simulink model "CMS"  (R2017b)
settings: Solver=FixedStepDiscrete  StartTime=0.0  StopTime=10.0  FixedStep=0.01  RelTol=1e-3  EnableMultiTasking=on
undefined symbols (not defined in the file): ASWTYPE_FALSE, ASWTYPE_TRUE, CcCMS_CANSendDelay_ms, CcCMS_ChrgMaxPackVoltLimt_V, CcCMS_PeakVoltCh_V, CcCMS_PeakVoltDisCh_V, CcSOC_DispSOCHighThrhd_pct, CMS09D_RUNTIME_MS, CMS_CONST0_NUMB, CMS_CONST1000_NUMB, CMS_CONST100_NUMB, CMS_CONST1_NUMB, CMS_CONST2047_NUMB, CMS_CONST2_NUMB, CMS_CONST3_NUMB, CMS_CONST4_NUMB, CMS_CONST5_NUMB, CMS_CONST6_NUMB, CMS_CONST7_NUMB, CMS_CONSTF1_NUMB, Enum_ACCACChrgState, Enum_CMSACChgMode, Enum_CMSBmsSelfChk, Enum_CMSBmsSt, Enum_CMSChgMode, Enum_CMSDCChgMode, Enum_CMSHVBatFltSevrtyStat, Enum_CMSHVConnSt, Enum_CMSPreThmMode, Enum_CMSPreThmReq, Enum_CMSThmPropagation, Enum_CTCCtrCtlConnMode, Enum_CTCCtrCtlState, Enum_DCCDCChrgState, Enum_DCCDCConnSt, Enum_ISOHVIsoFltLevel, Enum_MSMBMUState, Enum_ODPCCState, Enum_VDPPreThmEna
libraries: AIWAYS_Powertrain_BMS_lib x148
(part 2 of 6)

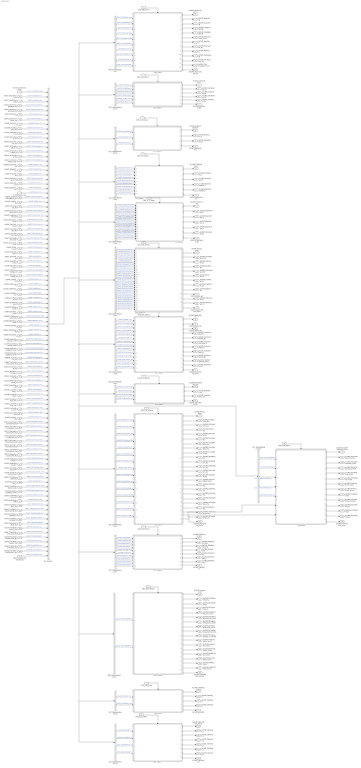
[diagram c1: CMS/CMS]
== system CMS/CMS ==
  CMS_09D_10ms : Inport
  CMS_2C0_100ms : Inport  Port=2
  CMS_2C2_100ms : Inport  Port=3
  CMS_2C3_100ms : Inport  Port=4
  CMS_2C7_100ms : Inport  Port=5
  CMS_2C8_100ms : Inport  Port=6
  CMS_2CA_100ms : Inport  Port=7
  CMS_2CD_100ms : Inport  Port=8
  CMS_2CE_100ms : Inport  Port=9
  CMS_2CF_100ms : Inport  Port=10
  CMS_3B0_1000ms : Inport  Port=11
  CMS_3E0_20ms : Inport  Port=12
  CMS_3E1_100ms : Inport  Port=13
  CMS_318_500ms : Inport  Port=14
  GeCTC_CtrCtlState_enum : Inport  Port=15
  GbCTC_NegCtlState_flg : Inport  Port=16
  GbCTC_PosCtlState_flg : Inport  Port=17
  GbCTC_DCPosChrgCtlState_flg : Inport  Port=18
  GbCTC_DCNegChrgCtlState_flg : Inport  Port=19
  GcHDP_PackVolt_V : Inport  Port=20
  GbCTC_PreChrgCtlState_flg : Inport  Port=21
  GcHDP_PackCrnt_A : Inport  Port=22
  GbWSM_Kl15WkUpPrs_flg : Inport  Port=23
  GcCDP_MinCellVolt_mV : Inport  Port=24
  GcCDP_MaxCellVolt_mV : Inport  Port=25
  GbACC_ObcChrgCmd_flg : Inport  Port=26
  GcACC_ACChrgVoltRqst_V : Inport  Port=27
  GcACC_ACChrgCrntRqst_A : Inport  Port=28
  GbACC_ACChrgRqst_flg : Inport  Port=29
  GeCTC_CtrCtlConnMode_enum : Inport  Port=30
  GbMSM_SelfCheck_flg : Inport  Port=31
  GcSOC_DispSOC_pct : Inport  Port=32
  GbISP_TFHvilLFlt_flg : Inport  Port=33
  GbFTC_OpenContactor_flg : Inport  Port=34
  GcSOH_PackSOH_pct : Inport  Port=35
  GcSOC_PackSOC_pct : Inport  Port=36
  GcHDP_HallCrnt_A : Inport  Port=37
  GbMSM_SelfChckMaxTiReach_flg : Inport  Port=38
  GaCDP_CellBalc_flg : Inport  Port=39
  GbDCC_DCChrgRqst_flg : Inport  Port=40
  GcSOP_DischrgConstPwr_kW : Inport  Port=41
  GcSOP_ChrgConstPwr_kW : Inport  Port=42
  GcISO_HVIsoValue_kohm : Inport  Port=43
  GeODP_ObcCcSt_enum : Inport  Port=44
  GbDCC_DCChrgFinish_flg : Inport  Port=45
  GbACC_ACChrgFinish_flg : Inport  Port=46
  GeACC_ACChrgState_enum : Inport  Port=47
  GeDCC_DCConnSt_enum : Inport  Port=48
  GeLDP_CC2St_enum : Inport  Port=49
  GcCDP_AvgCellTemp_C : Inport  Port=50
  GbISO_IsoForbid_flg : Inport  Port=51
  GcCDP_MaxCellTemp_C : Inport  Port=52
  GcCDP_MinCellTemp_C : Inport  Port=53
  GcDCS_3072ChrgVoltReq_V : Inport  Port=54
  GcDCC_DCChrgCrntRqst_A : Inport  Port=55
  GaCDP_CellVolt_mV : Inport  Port=56
  GaCDP_CellTemp_C : Inport  Port=57
  GcLDP_lntWtTemp_C : Inport  Port=58
  GcLDP_OutWtTemp_C : Inport  Port=59
  GcBTM_CoolPwrReq_W : Inport  Port=60
  GcBTM_HeatPwrReq_W : Inport  Port=61
  GeBTM_CoolReq_enum : Inport  Port=62
  GeBTM_HeatReq_enum : Inport  Port=63
  GbODP_V2XDischrgCmd_flg : Inport  Port=64
  GeMSM_BMUState_enum : Inport  Port=65
  GcHDP_FuseVolt_V : Inport  Port=66
  GbADP_DischgReq_flg : Inport  Port=67
  GcHDP_PosCtlVolt_V : Inport  Port=68
  GcCDP_MaxCellVoltNumb_numb : Inport  Port=69
  GcCDP_MinCellVoltNumb_numb : Inport  Port=70
  GcCDP_MaxCellTempNumb_numb : Inport  Port=71
  GcCDP_MinCellTempNumb_numb : Inport  Port=72
  GbWSM_DCWkUpPrs_flg : Inport  Port=73
  GbACC_PreThmObcChrgCmd_flg : Inport  Port=74
  GbACC_PreThmRqst_flg : Inport  Port=75
  GcACC_PreThmCrntRqst_A : Inport  Port=76
  GcACC_PreThmVoltRqst_V : Inport  Port=77
  GbACC_PreHeatPrmt_flg : Inport  Port=78
  GbFTC_PowerDown_flg : Inport  Port=79
  GcBTM_CoolTempReq_C : Inport  Port=80
  GcBTM_HeatTempReq_C : Inport  Port=81
  GcACC_ChrgingTiRem_min : Inport  Port=82
  GcDCC_ChrgingTiRem_min : Inport  Port=83
  GeVDP_PreThmEna_enum : Inport  Port=84
  GcSOP_DischrgPwr_kW : Inport  Port=85
  GcSOP_ChrgPwr_kW : Inport  Port=86
  GbFTC_DischrgPwrLimitLevel3_flg : Inport  Port=87
  GbFTC_RegenPwrLimitLevel3_flg : Inport  Port=88
  GbFTC_DischrgPwrLimitLevel2_flg : Inport  Port=89
  GbFTC_RegenPwrLimitLevel2_flg : Inport  Port=90
  GbFTC_DCChrgCurrLimitLevel2_flg : Inport  Port=91
  GbFTC_ACChrgCurrLimitLevel2_flg : Inport  Port=92
  GbFTC_DischrgPwrLimitLevel1_flg : Inport  Port=93
  GbFTC_RegenPwrLimitLevel1_flg : Inport  Port=94
  GcCDP_MaxBusbarTemp_C : Inport  Port=95
  GcCDP_MinBusbarTemp_C : Inport  Port=96
  GeDCC_DCChrgState_enum : Inport  Port=97
  GeLDP_ChrgGunConnSt_enum : Inport  Port=98
  GbISP_TFThmRnwyfDet_flg : Inport  Port=99
  GaCDP_BusbarTemp_C : Inport  Port=100
  GcUDS_CellTempNumb_numb : Inport  Port=101
  GcUDS_BusbarTempNumb_numb : Inport  Port=102
  GcUDS_CellVoltNum_numb : Inport  Port=103
  GcUDS_BatEnergy_kWh : Inport  Port=104
  GbACC_HoldTempPrmt_flg : Inport  Port=105
  GbACC_HoldTempObcChrgCmd_flg : Inport  Port=106
  GcACC_HoldTempVoltRqst_V : Inport  Port=107
  GcACC_HoldTempCrntRqst_A : Inport  Port=108
  GbACC_HoldTempRqst_flg : Inport  Port=109
  GbISP_TFIsoResFltLevel2_flg : Inport  Port=110
  GbISP_TFIsoDCResFltLevel2_flg : Inport  Port=111
  GbISP_TFIsoHVoffResFltLevel2_flg : Inport  Port=112
  GbISP_TFIsoResFltLevel1_flg : Inport  Port=113
  GbISP_TFIsoDCResFltLevel1_flg : Inport  Port=114
  GbISP_TFIsoHVoffResFltLevel1_flg : Inport  Port=115
  GbFTC_Level1FltReaction_flg : Inport  Port=116
  09D_10ms : Subsystem
  09D_10msBusSelector : BusSelector  OutputSignals=GeCTC_CtrCtlState_enum,GbCTC_NegCtlState_flg,GbCTC_PosCtlState_flg,GbCTC_DCPosChrgCtlState_flg,GbCTC_DCNegChrgCtlState_flg,GbCTC_PreChrgCtlState_flg,GcHDP_PackCrnt_A,GbWSM_Kl15WkUpPrs_flg,GcHDP_PosCtlVolt_V,GbISP_TFThmRnwyfDet_flg
  2C0_100ms : Subsystem
  2C0_100msBusSelector : BusSelector  OutputSignals=GcLDP_lntWtTemp_C,GcLDP_OutWtTemp_C,GcBTM_CoolPwrReq_W,GcBTM_HeatPwrReq_W,GeBTM_CoolReq_enum,GeBTM_HeatReq_enum
  2C2_100ms : Subsystem
  2C3_100ms : Subsystem
  2C3_100msBusSelector : BusSelector  OutputSignals=GcCDP_MinCellVolt_mV,GcCDP_MaxCellVolt_mV,GcBTM_CoolTempReq_C,GcBTM_HeatTempReq_C,GcCDP_MaxBusbarTemp_C,GcCDP_MinBusbarTemp_C,GcUDS_BusbarTempNumb_numb,GcCDP_MaxCellTemp_C,GcCDP_MinCellTemp_C
  2C3_100msBusSelector1 : BusSelector  OutputSignals=GcSOP_DischrgPwr_kW,GcSOP_ChrgPwr_kW,GcHDP_PackVolt_V
  2C7_100ms : Subsystem
  2C7_100msBusSelector : BusSelector  OutputSignals=GbACC_ObcChrgCmd_flg,GcHDP_PackVolt_V,GcHDP_PackCrnt_A,GcACC_ACChrgVoltRqst_V,GcACC_ACChrgCrntRqst_A,GbACC_ACChrgRqst_flg,GbODP_V2XDischrgCmd_flg,GbACC_PreThmObcChrgCmd_flg,GcACC_PreThmCrntRqst_A,GcACC_PreThmVoltRqst_V,GbACC_PreHeatPrmt_flg,GbACC_HoldTempObcChrgCmd_flg,GbACC_HoldTempPrmt_flg,GcACC_HoldTempVoltRqst_V,GcACC_HoldTempCrntRqst_A
  2C8_100ms : Subsystem
  2C8_100msBusSelector : BusSelector  OutputSignals=GeCTC_CtrCtlConnMode_enum,GbMSM_SelfCheck_flg,GcSOC_DispSOC_pct,GbISP_TFHvilLFlt_flg,GcSOH_PackSOH_pct,GcHDP_HallCrnt_A,GbMSM_SelfChckMaxTiReach_flg,GeCTC_CtrCtlState_enum,GeMSM_BMUState_enum,GeODP_ObcCcSt_enum,GeVDP_PreThmEna_enum,GbFTC_OpenContactor_flg,GbFTC_PowerDown_flg,GbFTC_DischrgPwrLimitLevel3_flg,GbFTC_RegenPwrLimitLevel3_flg,GbFTC_DischrgPwrLimitLevel2_flg,GbFTC_RegenPwrLimitLevel2_flg,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
  2CA_100ms : Subsystem
  2CA_100msBusSelector : BusSelector  OutputSignals=GaCDP_CellBalc_flg,GbDCC_DCChrgRqst_flg,GbACC_ACChrgRqst_flg,GeCTC_CtrCtlConnMode_enum,GbADP_DischgReq_flg,GcHDP_PackVolt_V,GbACC_PreThmRqst_flg,GbFTC_PowerDown_flg,GbACC_PreHeatPrmt_flg,GeVDP_PreThmEna_enum,GcSOP_DischrgConstPwr_kW,GcSOP_ChrgConstPwr_kW,GbACC_HoldTempPrmt_flg,GbACC_HoldTempRqst_flg
  2CD_100ms : Subsystem
  2CD_100msBusSelector : BusSelector  OutputSignals=GcSOP_DischrgPwr_kW,GcSOP_ChrgPwr_kW,GcSOP_DischrgConstPwr_kW,GcSOP_ChrgConstPwr_kW
  2CE_100ms : Subsystem
  2CE_100msBusSelector : BusSelector  OutputSignals=GcISO_HVIsoValue_kohm,GeODP_ObcCcSt_enum,GbDCC_DCChrgFinish_flg,GbACC_ACChrgFinish_flg,GcSOC_PackSOC_pct,GeACC_ACChrgState_enum,GeDCC_DCConnSt_enum,GeLDP_CC2St_enum,GcACC_ChrgingTiRem_min,GcDCC_ChrgingTiRem_min,GeCTC_CtrCtlConnMode_enum,GbACC_PreHeatPrmt_flg,GeVDP_PreThmEna_enum,GeDCC_DCChrgState_enum,GeLDP_ChrgGunConnSt_enum
  2CF_100ms : Subsystem
  2CF_100msBusSelector : BusSelector  OutputSignals=GcCDP_AvgCellTemp_C,GbISO_IsoForbid_flg,GcCDP_MaxCellTemp_C,GcCDP_MinCellTemp_C,GcSOC_DispSOC_pct,GcHDP_FuseVolt_V,GcUDS_BatEnergy_kWh,GcUDS_CellTempNumb_numb,GcCDP_MaxBusbarTemp_C,GcCDP_MinBusbarTemp_C
  2CF_100msBusSelector1 : BusSelector  OutputSignals=GaCDP_CellVolt_mV,GcUDS_CellVoltNum_numb
  2CF_100msBusSelector2 : BusSelector  OutputSignals=GaCDP_CellTemp_C,GaCDP_BusbarTemp_C,GcUDS_CellTempNumb_numb,GcUDS_BusbarTempNumb_numb
  2CF_100msBusSelector3 : BusSelector  OutputSignals=GcCDP_MaxCellVoltNumb_numb,GcCDP_MinCellVoltNumb_numb,GcCDP_MaxCellTempNumb_numb,GcCDP_MinCellTempNumb_numb,GbWSM_DCWkUpPrs_flg
  318_500ms : Subsystem
  3B0_1000ms : Subsystem
  3B0_1000msBusSelector : BusSelector  OutputSignals=GcDCS_3072ChrgVoltReq_V,GcDCC_DCChrgCrntRqst_A
  3E0_20ms : Subsystem
  3E1_100ms : Subsystem
  Bus Creator : BusCreator  Inputs=102
  GeCMS_HVConnSt_enum : Outport
  GbCMS_NegCtlSt_flg : Outport  Port=2
  GbCMS_PosCtlSt_flg : Outport  Port=3
  GbCMS_ChrgPosCtlSt_flg : Outport  Port=4
  GbCMS_ChrgNegCtlSt_flg : Outport  Port=5
  GeCMS_RelStuckClosed_enum : Outport  Port=6
  GcCMS_PackVolt_V : Outport  Port=7
  GbCMS_PreChrgCtlSt_flg : Outport  Port=8
  GcCMS_BattCurr_A : Outport  Port=9
  GbCMS_Kl15WkUp_flg : Outport  Port=10
  GbCMS_ThmRunAway_flg : Outport  Port=11
  GcCMS_CoolTempIn_C : Outport  Port=12
  GcCMS_CoolTempOut_C : Outport  Port=13
  GcCMS_CoolPwrReq_W : Outport  Port=14
  GcCMS_HeatPwrReq_W : Outport  Port=15
  GeCMS_CoolReq_enum : Outport  Port=16
  GeCMS_HeatReq_enum : Outport  Port=17
  GcCMS_PeakCurrDisCh_A : Outport  Port=18
  GcCMS_PeakCurrCh_A : Outport  Port=19
  GcCMS_PeakVoltDisCh_V : Outport  Port=20
  GcCMS_PeakVoltCh_V : Outport  Port=21
  GcCMS_ClntTgtTemp_C : Outport  Port=22
  GcCMS_HtTgtTemp_C : Outport  Port=23
  GcCMS_MaxCellVolt_V : Outport  Port=24
  GcCMS_BusbarTempMax_C : Outport  Port=25
  GcCMS_BusbarTempMin_C : Outport  Port=26
  GcCMS_MinCellVolt_V : Outport  Port=27
  GbCMS_ChrgCmd_flg : Outport  Port=28
  GcCMS_ActPwrChrg_Kw : Outport  Port=29
  GcCMS_MaxVoltChrg_V : Outport  Port=30
  GcCMS_ReqVoltChrg_V : Outport  Port=31
  GcCMS_ReqCurrChrg_A : Outport  Port=32
  GbCMS_ObcRdyReq_flg : Outport  Port=33
  GbCMS_DischgCmd_flg : Outport  Port=34
  GeCMS_BmsSt_enum : Outport  Port=35
  GeCMS_BmsSelfChk_enum : Outport  Port=36
  GeCMS_IsoFault_enum : Outport  Port=37
  GcCMS_SocDspl_pct : Outport  Port=38
  GbCMS_HvilOpenFault_flg : Outport  Port=39
  GeCMS_FltLvl_enum : Outport  Port=40
  GeCMS_V2xMod_enum : Outport  Port=41
  GcCMS_ChgSOCset_pct : Outport  Port=42
  GcCMS_BattSoh_pct : Outport  Port=43
  GcCMS_SOCA_pct : Outport  Port=44
  GeCMS_IviDischg_enum : Outport  Port=45
  GcCMS_PackCurLem_A : Outport  Port=46
  GcCMS_BattInVolt_V : Outport  Port=47
  GbCMS_BalSt_flg : Outport  Port=48
  GbCMS_BalVlg_flg : Outport  Port=49
  GbCMS_VcuPwrUpReq_flg : Outport  Port=50
  GbCMS_VcuPwrUpReqVld_flg : Outport  Port=51
  GcCMS_ConstCurrDisChMax_A : Outport  Port=52
  GcCMS_ConstCurrChMax_A : Outport  Port=53
  GbCMS_PwrDownReq_flg : Outport  Port=54
  GbCMS_PwrDownReqVld_flg : Outport  Port=55
  GeCMS_ChrgPreThmMode_enum : Outport  Port=56
  GeCMS_ElockReq_enum : Outport  Port=57
  GeCMS_PreThmReq_enum : Outport  Port=58
  GcCMS_PeakPwrDisCh_Kw : Outport  Port=59
  GcCMS_PeakPwrCh_Kw : Outport  Port=60
  GcCMS_ConstPwrDisCh_Kw : Outport  Port=61
  GcCMS_ConstPwrCh_Kw : Outport  Port=62
  GcCMS_ResIso_Kohm : Outport  Port=63
  GcCMS_ChrgRemTime_Min : Outport  Port=64
  GeCMS_ACPlugCnnt_enum : Outport  Port=65
  GbCMS_BattFull_flg : Outport  Port=66
  GbCMS_WarnLamp_flg : Outport  Port=67
  GbCMS_SerLamp_flg : Outport  Port=68
  GbCMS_TempDiffWarn_flg : Outport  Port=69
  GbCMS_OverChrgWarn_flg : Outport  Port=70
  GbCMS_ConsisWarn_flg : Outport  Port=71
  GbCMS_MishWarn_flg : Outport  Port=72
  GbCMS_SocHopWarn_flg : Outport  Port=73
  GbCMS_SocHighWarn_flg : Outport  Port=74
  GbCMS_SocLowWarn_flg : Outport  Port=75
  GbCMS_OTAModeSt_flg : Outport  Port=76
  GeCMS_AcDcConnBoth_enum : Outport  Port=77
  GbCMS_CellUvFlt_flg : Outport  Port=78
  GbCMS_CellOvFlt_flg : Outport  Port=79
  GbCMS_PackUvFlt_flg : Outport  Port=80
  GbCMS_PackOvFlt_flg : Outport  Port=81
  GbCMS_TempHighWarn_flg : Outport  Port=82
  GcCMS_RealSoc_pct : Outport  Port=83
  GeCMS_DCPlugConn_enum : Outport  Port=84
  GeCMS_ACChgMode_enum : Outport  Port=85
  GeCMS_DCChgMode_enum : Outport  Port=86
  GcCMS_BattTempAvrg_C : Outport  Port=87
  GcCMS_BattNrmEnrg_kwh : Outport  Port=88
  GbCMS_BattTempFault_flg : Outport  Port=89
  GcCMS_BattSoe_kwh : Outport  Port=90
  GbCMS_IsoChkSt_flg : Outport  Port=91
  GcCMS_BattTempMax_C : Outport  Port=92
  GcCMS_BattTempMin_C : Outport  Port=93
  GcCMS_FuseVolt_V : Outport  Port=94
  GcCMS_ChrgAccum_Ah : Outport  Port=95
  GbCMS_DChgStVoltOut_flg : Outport  Port=96
  GcCMS_DChrgVoltReq_V : Outport  Port=97
  GcCMS_DChrgCurrReq_A : Outport  Port=98
  GcCMS_DChrgRchSocLmt_numb : Outport  Port=99
  GcCMS_DChrgRchPackVoltLmt_numb : Outport  Port=100
  GcCMS_DChrgRchCellVoltLmt_numb : Outport  Port=101
  GcCMS_DChrgChrgerActStop_numb : Outport  Port=102
  GcCMS_DChrgBattInsulationErr_numb : Outport  Port=103
  GcCMS_DChrgOutpCnntOvrTempErr_numb : Outport  Port=104
  GcCMS_PcbOvrTempErr_numb : Outport  Port=105
  GcCMS_ChrgCnntErr_numb : Outport  Port=106
  GcCMS_BattOvrTempErr_numb : Outport  Port=107
  GcCMS_MainRelayErr_numb : Outport  Port=108
  GcCMS_CC2ChkVoltErr_numb : Outport  Port=109
  GcCMS_OtherErr_numb : Outport  Port=110
  GcCMS_ChrgCurrAbnrm_numb : Outport  Port=111
  GcCMS_ChrgVoltAbnrm_numb : Outport  Port=112
  GcCMS_CellVoltCnt_numb : Outport  Port=113
  GcCMS_CellVolt1_V : Outport  Port=114
  GcCMS_CellVolt2_V : Outport  Port=115
  GcCMS_CellVolt3_V : Outport  Port=116
  GcCMS_CellVolt4_V : Outport  Port=117
  GcCMS_CellTempCnt_numb : Outport  Port=118
  GcCMS_CellTemp1_C : Outport  Port=119
  GcCMS_CellTemp2_C : Outport  Port=120
  GcCMS_CellTemp3_C : Outport  Port=121
  GcCMS_CellTemp4_C : Outport  Port=122
  GcCMS_CellTemp5_C : Outport  Port=123
  GcCMS_CellTemp6_C : Outport  Port=124
  GcCMS_CellTemp7_C : Outport  Port=125
  GcCMS_MaxCellVoltNumb_numb : Outport  Port=126
  GcCMS_MinCellVoltNumb_numb : Outport  Port=127
  GcCMS_MaxCellTempNumb_numb : Outport  Port=128
  GcCMS_MinCellTempNumb_numb : Outport  Port=129
  GcCMS_MaxVoltNumb_numb : Outport  Port=130
  GcCMS_MinVoltNumb_numb : Outport  Port=131
  GcCMS_MaxTempNumb_numb : Outport  Port=132
  GcCMS_MinTempNumb_numb : Outport  Port=133
  GeCMS_ChgMode_enum : Outport  Port=134
  GeCMS_DChrgModeDebug_enum : Outport  Port=135
  GbCMS_DChrgWkUp_flg : Outport  Port=136
  GeCMS_EvccMode_enum : Outport  Port=137
  GeCMS_AChrgObsr_enum : Outport  Port=138
  GeCMS_PreThmObsvr_enum : Outport  Port=139
  GeCMS_Thm_propagat_enum : Outport  Port=140
  GbCMS_StartCanSend_flg : Outport  Port=141
  GeCMS_AppChgMode_enum : Outport  Port=142
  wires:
  CMS_09D_10ms/1 -> 09D_10ms/Trigger
  CMS_2C0_100ms/1 -> 2C0_100ms/Trigger
  CMS_2C2_100ms/1 -> 2C2_100ms/Trigger
  CMS_2C3_100ms/1 -> 2C3_100ms/Trigger
  CMS_2C7_100ms/1 -> 2C7_100ms/Trigger
  CMS_2C8_100ms/1 -> 2C8_100ms/Trigger
  CMS_2CA_100ms/1 -> 2CA_100ms/Trigger
  CMS_2CD_100ms/1 -> 2CD_100ms/Trigger
  CMS_2CE_100ms/1 -> 2CE_100ms/Trigger
  CMS_2CF_100ms/1 -> 2CF_100ms/Trigger
  CMS_3B0_1000ms/1 -> 3B0_1000ms/Trigger
  CMS_3E0_20ms/1 -> 3E0_20ms/Trigger
  CMS_3E1_100ms/1 -> 3E1_100ms/Trigger
  CMS_318_500ms/1 -> 318_500ms/Trigger
  09D_10msBusSelector/1 -> 09D_10ms/1(GeCTC_CtrCtlState_enum)  "<GeCTC_CtrCtlState_enum>"
  09D_10msBusSelector/2 -> 09D_10ms/2(GbCTC_NegCtlState_flg)  "<GbCTC_NegCtlState_flg>"
  09D_10msBusSelector/3 -> 09D_10ms/3(GbCTC_PosCtlState_flg)  "<GbCTC_PosCtlState_flg>"
  09D_10msBusSelector/4 -> 09D_10ms/4(GbCTC_DCPosChrgCtlState_flg)  "<GbCTC_DCPosChrgCtlState_flg>"
  09D_10msBusSelector/5 -> 09D_10ms/5(GbCTC_DCNegChrgCtlState_flg)  "<GbCTC_DCNegChrgCtlState_flg>"
  09D_10msBusSelector/6 -> 09D_10ms/6(GbCTC_PreChrgCtlState_flg)  "<GbCTC_PreChrgCtlState_flg>"
  09D_10msBusSelector/7 -> 09D_10ms/7(GcHDP_PackCrnt_A)  "<GcHDP_PackCrnt_A>"
  09D_10msBusSelector/8 -> 09D_10ms/8(GbWSM_Kl15WkUpPrs_flg)  "<GbWSM_Kl15WkUpPrs_flg>"
  09D_10ms/1(GeCMS_HVConnSt_enum) -> GeCMS_HVConnSt_enum/1
  09D_10ms/2(GbCMS_NegCtlSt_flg) -> GbCMS_NegCtlSt_flg/1
  09D_10ms/3(GbCMS_PosCtlSt_flg) -> GbCMS_PosCtlSt_flg/1
  09D_10ms/4(GbCMS_ChrgPosCtlSt_flg) -> GbCMS_ChrgPosCtlSt_flg/1
  09D_10ms/5(GbCMS_ChrgNegCtlSt_flg) -> GbCMS_ChrgNegCtlSt_flg/1
  09D_10ms/6(GeCMS_RelStuckClosed_enum) -> GeCMS_RelStuckClosed_enum/1
  09D_10ms/7(GcCMS_PackVolt_V) -> GcCMS_PackVolt_V/1
  09D_10ms/8(GbCMS_PreChrgCtlSt_flg) -> GbCMS_PreChrgCtlSt_flg/1
  09D_10ms/9(GcCMS_BattCurr_A) -> GcCMS_BattCurr_A/1
  09D_10ms/10(GbCMS_Kl15WkUp_flg) -> GbCMS_Kl15WkUp_flg/1
  09D_10ms/11(GbCMS_ThmRunAway_flg) -> GbCMS_ThmRunAway_flg/1
  2C0_100msBusSelector/1 -> 2C0_100ms/1(GcLDP_lntWtTemp_C)  "<GcLDP_lntWtTemp_C>"
  2C0_100msBusSelector/2 -> 2C0_100ms/2(GcLDP_OutWtTemp_C)  "<GcLDP_OutWtTemp_C>"
  2C0_100msBusSelector/3 -> 2C0_100ms/3(GcBTM_CoolPwrReq_W)  "<GcBTM_CoolPwrReq_W>"
  2C0_100msBusSelector/4 -> 2C0_100ms/4(GcBTM_HeatPwrReq_W)  "<GcBTM_HeatPwrReq_W>"
  2C0_100msBusSelector/5 -> 2C0_100ms/5(GeBTM_CoolReq_enum)  "<GeBTM_CoolReq_enum>"
  2C0_100msBusSelector/6 -> 2C0_100ms/6(GeBTM_HeatReq_enum)  "<GeBTM_HeatReq_enum>"
  2C0_100ms/1(GcCMS_CoolTempIn_C) -> GcCMS_CoolTempIn_C/1
  2C0_100ms/2(GcCMS_CoolTempOut_C) -> GcCMS_CoolTempOut_C/1
  2C0_100ms/3(GcCMS_CoolPwrReq_W) -> GcCMS_CoolPwrReq_W/1
  2C0_100ms/4(GcCMS_HeatPwrReq_W) -> GcCMS_HeatPwrReq_W/1
  2C0_100ms/5(GeCMS_CoolReq_enum) -> GeCMS_CoolReq_enum/1
  2C0_100ms/6(GeCMS_HeatReq_enum) -> GeCMS_HeatReq_enum/1
  2C2_100ms/1(GcCMS_PeakCurrDisCh_A) -> GcCMS_PeakCurrDisCh_A/1
  2C2_100ms/2(GcCMS_PeakCurrCh_A) -> GcCMS_PeakCurrCh_A/1
  2C2_100ms/3(GcCMS_PeakVoltDisCh_V) -> GcCMS_PeakVoltDisCh_V/1
  2C2_100ms/4(GcCMS_PeakVoltCh_V) -> GcCMS_PeakVoltCh_V/1
  2C3_100msBusSelector/1 -> 2C3_100ms/1(GcCDP_MinCellVolt_mV)  "<GcCDP_MinCellVolt_mV>"
  2C3_100msBusSelector/2 -> 2C3_100ms/2(GcCDP_MaxCellVolt_mV)  "<GcCDP_MaxCellVolt_mV>"
  2C3_100ms/1(GcCMS_ClntTgtTemp_C) -> GcCMS_ClntTgtTemp_C/1
  2C3_100ms/2(GcCMS_HtTgtTemp_C) -> GcCMS_HtTgtTemp_C/1
  2C3_100ms/3(GcCMS_MaxCellVolt_V) -> GcCMS_MaxCellVolt_V/1
  2C3_100ms/4(GcCMS_BusbarTempMax_C) -> GcCMS_BusbarTempMax_C/1
  2C3_100ms/5(GcCMS_BusbarTempMin_C) -> GcCMS_BusbarTempMin_C/1
  2C3_100ms/6(GcCMS_MinCellVolt_V) -> GcCMS_MinCellVolt_V/1
  2C7_100msBusSelector/1 -> 2C7_100ms/1(GbACC_ObcChrgCmd_flg)  "<GbACC_ObcChrgCmd_flg>"
  2C7_100msBusSelector/2 -> 2C7_100ms/2(GcHDP_PackVolt_V)  "<GcHDP_PackVolt_V>"
  2C7_100msBusSelector/3 -> 2C7_100ms/3(GcHDP_PackCrnt_A)  "<GcHDP_PackCrnt_A>"
  2C7_100msBusSelector/4 -> 2C7_100ms/4(GcACC_ACChrgVoltRqst_V)  "<GcACC_ACChrgVoltRqst_V>"
  2C7_100msBusSelector/5 -> 2C7_100ms/5(GcACC_ACChrgCrntRqst_A)  "<GcACC_ACChrgCrntRqst_A>"
  2C7_100msBusSelector/6 -> 2C7_100ms/6(GbACC_ACChrgRqst_flg)  "<GbACC_ACChrgRqst_flg>"
  2C7_100ms/1(GbCMS_ChrgCmd_flg) -> GbCMS_ChrgCmd_flg/1
  2C7_100ms/2(GcCMS_ActPwrChrg_Kw) -> GcCMS_ActPwrChrg_Kw/1
  2C7_100ms/3(GcCMS_MaxVoltChrg_V) -> GcCMS_MaxVoltChrg_V/1
  2C7_100ms/4(GcCMS_ReqVoltChrg_V) -> GcCMS_ReqVoltChrg_V/1
  2C7_100ms/5(GcCMS_ReqCurrChrg_A) -> GcCMS_ReqCurrChrg_A/1
  2C7_100ms/6(GbCMS_ObcRdyReq_flg) -> GbCMS_ObcRdyReq_flg/1
  2C7_100ms/7(GbCMS_DischgCmd_flg) -> GbCMS_DischgCmd_flg/1
  2C8_100msBusSelector/1 -> 2C8_100ms/1(GeCTC_CtrCtlConnMode_enum)  "<GeCTC_CtrCtlConnMode_enum>"
  2C8_100msBusSelector/2 -> 2C8_100ms/2(GbMSM_SelfCheck_flg)  "<GbMSM_SelfCheck_flg>"
  2C8_100msBusSelector/3 -> 2C8_100ms/3(GcSOC_DispSOC_pct)  "<GcSOC_DispSOC_pct>"
  2C8_100msBusSelector/4 -> 2C8_100ms/4(GbISP_TFHvilLFlt_flg)  "<GbISP_TFHvilLFlt_flg>"
  2C8_100msBusSelector/5 -> 2C8_100ms/5(GcSOH_PackSOH_pct)  "<GcSOH_PackSOH_pct>"
  2C8_100msBusSelector/6 -> 2C8_100ms/6(GcHDP_HallCrnt_A)  "<GcHDP_HallCrnt_A>"
  2C8_100msBusSelector/7 -> 2C8_100ms/7(GbMSM_SelfChckMaxTiReach_flg)  "<GbMSM_SelfChckMaxTiReach_flg>"
  2C8_100ms/1(GeCMS_BmsSt_enum) -> GeCMS_BmsSt_enum/1
  2C8_100ms/2(GeCMS_BmsSelfChk_enum) -> GeCMS_BmsSelfChk_enum/1
  2C8_100ms/3(GeCMS_IsoFault_enum) -> GeCMS_IsoFault_enum/1
  2C8_100ms/4(GcCMS_SocDspl_pct) -> GcCMS_SocDspl_pct/1
  2C8_100ms/5(GbCMS_HvilOpenFault_flg) -> GbCMS_HvilOpenFault_flg/1
  2C8_100ms/6(GeCMS_FltLvl_enum) -> GeCMS_FltLvl_enum/1
  2C8_100ms/7(GeCMS_V2xMod_enum) -> GeCMS_V2xMod_enum/1
  2C8_100ms/8(GcCMS_ChgSOCset_pct) -> GcCMS_ChgSOCset_pct/1
  2C8_100ms/9(GcCMS_BattSoh_pct) -> GcCMS_BattSoh_pct/1
  2C8_100ms/10(GcCMS_SOCA_pct) -> GcCMS_SOCA_pct/1
  2C8_100ms/11(GeCMS_IviDischg_enum) -> GeCMS_IviDischg_enum/1
  2C8_100ms/12(GcCMS_PackCurLem_A) -> GcCMS_PackCurLem_A/1
  2CA_100msBusSelector/1 -> 2CA_100ms/1(GaCDP_CellBalc_flg)  "<GaCDP_CellBalc_flg>"
  2CA_100msBusSelector/2 -> 2CA_100ms/2(GbDCC_DCChrgRqst_flg)  "<GbDCC_DCChrgRqst_flg>"
  2CA_100msBusSelector/3 -> 2CA_100ms/3(GbACC_ACChrgRqst_flg)  "<GbACC_ACChrgRqst_flg>"
  2CA_100msBusSelector/4 -> 2CA_100ms/4(GeCTC_CtrCtlConnMode_enum)  "<GeCTC_CtrCtlConnMode_enum>"
  2CA_100ms/1(GcCMS_BattInVolt_V) -> GcCMS_BattInVolt_V/1
  2CA_100ms/2(GbCMS_BalSt_flg) -> GbCMS_BalSt_flg/1
  2CA_100ms/3(GbCMS_BalVlg_flg) -> GbCMS_BalVlg_flg/1
  2CA_100ms/4(GbCMS_VcuPwrUpReq_flg) -> GbCMS_VcuPwrUpReq_flg/1
  2CA_100ms/5(GbCMS_VcuPwrUpReqVld_flg) -> GbCMS_VcuPwrUpReqVld_flg/1
  2CA_100ms/6(GcCMS_ConstCurrDisChMax_A) -> GcCMS_ConstCurrDisChMax_A/1
  2CA_100ms/7(GcCMS_ConstCurrChMax_A) -> GcCMS_ConstCurrChMax_A/1
  2CA_100ms/8(GbCMS_PwrDownReq_flg) -> GbCMS_PwrDownReq_flg/1
  2CA_100ms/9(GbCMS_PwrDownReqVld_flg) -> GbCMS_PwrDownReqVld_flg/1
  2CA_100ms/10(GeCMS_ChrgPreThmMode_enum) -> GeCMS_ChrgPreThmMode_enum/1
  2CA_100ms/11(GeCMS_ElockReq_enum) -> GeCMS_ElockReq_enum/1
  2CA_100ms/12(GeCMS_PreThmReq_enum) -> GeCMS_PreThmReq_enum/1
  2CD_100msBusSelector/3 -> 2CD_100ms/3(GcSOP_DischrgConstPwr_kW)  "<GcSOP_DischrgConstPwr_kW>"
  2CD_100msBusSelector/4 -> 2CD_100ms/4(GcSOP_ChrgConstPwr_kW)  "<GcSOP_ChrgConstPwr_kW>"
  2CD_100ms/1(GcCMS_PeakPwrDisCh_Kw) -> GcCMS_PeakPwrDisCh_Kw/1
  2CD_100ms/2(GcCMS_PeakPwrCh_Kw) -> GcCMS_PeakPwrCh_Kw/1
  2CD_100ms/3(GcCMS_ConstPwrDisCh_Kw) -> GcCMS_ConstPwrDisCh_Kw/1
  2CD_100ms/4(GcCMS_ConstPwrCh_Kw) -> GcCMS_ConstPwrCh_Kw/1
  2CE_100msBusSelector/1 -> 2CE_100ms/1(GcISO_HVIsoValue_kohm)  "<GcISO_HVIsoValue_kohm>"
  2CE_100msBusSelector/2 -> 2CE_100ms/2(GeODP_ObcCcSt_enum)  "<GeODP_ObcCcSt_enum>"
  2CE_100msBusSelector/3 -> 2CE_100ms/3(GbDCC_DCChrgFinish_flg)  "<GbDCC_DCChrgFinish_flg>"
  2CE_100msBusSelector/4 -> 2CE_100ms/4(GbACC_ACChrgFinish_flg)  "<GbACC_ACChrgFinish_flg>"
  2CE_100msBusSelector/5 -> 2CE_100ms/5(GcSOC_PackSOC_pct)  "<GcSOC_PackSOC_pct>"
  2CE_100msBusSelector/6 -> 2CE_100ms/6(GeACC_ACChrgState_enum)  "<GeACC_ACChrgState_enum>"
  2CE_100msBusSelector/7 -> 2CE_100ms/7(GeDCC_DCConnSt_enum)  "<GeDCC_DCConnSt_enum>"
  2CE_100msBusSelector/8 -> 2CE_100ms/8(GeLDP_CC2St_enum)  "<GeLDP_CC2St_enum>"
  2CE_100ms/1(GcCMS_ResIso_Kohm) -> GcCMS_ResIso_Kohm/1
  2CE_100ms/2(GcCMS_ChrgRemTime_Min) -> GcCMS_ChrgRemTime_Min/1
  2CE_100ms/3(GeCMS_ACPlugCnnt_enum) -> GeCMS_ACPlugCnnt_enum/1
  2CE_100ms/4(GbCMS_BattFull_flg) -> GbCMS_BattFull_flg/1
  2CE_100ms/5(GbCMS_WarnLamp_flg) -> GbCMS_WarnLamp_flg/1
  2CE_100ms/6(GbCMS_SerLamp_flg) -> GbCMS_SerLamp_flg/1
  2CE_100ms/7(GbCMS_TempDiffWarn_flg) -> GbCMS_TempDiffWarn_flg/1
  2CE_100ms/8(GbCMS_OverChrgWarn_flg) -> GbCMS_OverChrgWarn_flg/1
  2CE_100ms/9(GbCMS_ConsisWarn_flg) -> GbCMS_ConsisWarn_flg/1
  2CE_100ms/10(GbCMS_MishWarn_flg) -> GbCMS_MishWarn_flg/1
  2CE_100ms/11(GbCMS_SocHopWarn_flg) -> GbCMS_SocHopWarn_flg/1
  2CE_100ms/12(GbCMS_SocHighWarn_flg) -> GbCMS_SocHighWarn_flg/1
  2CE_100ms/13(GbCMS_SocLowWarn_flg) -> GbCMS_SocLowWarn_flg/1
  2CE_100ms/14(GbCMS_OTAModeSt_flg) -> GbCMS_OTAModeSt_flg/1
  2CE_100ms/15(GeCMS_AcDcConnBoth_enum) -> GeCMS_AcDcConnBoth_enum/1
  2CE_100ms/16(GbCMS_CellUvFlt_flg) -> GbCMS_CellUvFlt_flg/1
  2CE_100ms/17(GbCMS_CellOvFlt_flg) -> GbCMS_CellOvFlt_flg/1
  2CE_100ms/18(GbCMS_PackUvFlt_flg) -> GbCMS_PackUvFlt_flg/1
  2CE_100ms/19(GbCMS_PackOvFlt_flg) -> GbCMS_PackOvFlt_flg/1
  2CE_100ms/20(GbCMS_TempHighWarn_flg) -> GbCMS_TempHighWarn_flg/1
  2CE_100ms/21(GcCMS_RealSoc_pct) -> GcCMS_RealSoc_pct/1
  2CE_100ms/22(GeCMS_DCPlugConn_enum) -> GeCMS_DCPlugConn_enum/1
  2CE_100ms/23(GeCMS_ACChgMode_enum) -> GeCMS_ACChgMode_enum/1, 318_500ms/6(GeCMS_ACChgMode_enum)
  2CE_100ms/24(GeCMS_DCChgMode_enum) -> 318_500ms/7(GeCMS_DCChgMode_enum), GeCMS_DCChgMode_enum/1
  2CF_100msBusSelector/1 -> 2CF_100ms/1(GcCDP_AvgCellTemp_C)  "<GcCDP_AvgCellTemp_C>"
  2CF_100msBusSelector/2 -> 2CF_100ms/2(GbISO_IsoForbid_flg)  "<GbISO_IsoForbid_flg>"
  2CF_100msBusSelector/3 -> 2CF_100ms/3(GcCDP_MaxCellTemp_C)  "<GcCDP_MaxCellTemp_C>"
  2CF_100msBusSelector/4 -> 2CF_100ms/4(GcCDP_MinCellTemp_C)  "<GcCDP_MinCellTemp_C>"
  2CF_100ms/1(GcCMS_BattTempAvrg_C) -> GcCMS_BattTempAvrg_C/1
  2CF_100ms/2(GcCMS_BattNrmEnrg_kwh) -> GcCMS_BattNrmEnrg_kwh/1
  2CF_100ms/3(GbCMS_BattTempFault_flg) -> GbCMS_BattTempFault_flg/1
  2CF_100ms/4(GcCMS_BattSoe_kwh) -> GcCMS_BattSoe_kwh/1
  2CF_100ms/5(GbCMS_IsoChkSt_flg) -> GbCMS_IsoChkSt_flg/1
  2CF_100ms/6(GcCMS_BattTempMax_C) -> GcCMS_BattTempMax_C/1
  2CF_100ms/7(GcCMS_BattTempMin_C) -> GcCMS_BattTempMin_C/1
  2CF_100ms/8(GcCMS_FuseVolt_V) -> GcCMS_FuseVolt_V/1
  3B0_1000msBusSelector/1 -> 3B0_1000ms/1(GcDCS_3072ChrgVoltReq_V)  "<GcDCS_3072ChrgVoltReq_V>"
  3B0_1000msBusSelector/2 -> 3B0_1000ms/2(GcDCC_DCChrgCrntRqst_A)  "<GcDCC_DCChrgCrntRqst_A>"
  3B0_1000ms/1(GcCMS_ChrgAccum_Ah) -> GcCMS_ChrgAccum_Ah/1
  3B0_1000ms/2(GbCMS_DChgStVoltOut_flg) -> GbCMS_DChgStVoltOut_flg/1
  3B0_1000ms/3(GcCMS_DChrgVoltReq_V) -> GcCMS_DChrgVoltReq_V/1
  3B0_1000ms/4(GcCMS_DChrgCurrReq_A) -> GcCMS_DChrgCurrReq_A/1
  3B0_1000ms/5(GcCMS_DChrgRchSocLmt_numb) -> GcCMS_DChrgRchSocLmt_numb/1
  3B0_1000ms/6(GcCMS_DChrgRchPackVoltLmt_numb) -> GcCMS_DChrgRchPackVoltLmt_numb/1
  3B0_1000ms/7(GcCMS_DChrgRchCellVoltLmt_numb) -> GcCMS_DChrgRchCellVoltLmt_numb/1
  3B0_1000ms/8(GcCMS_DChrgChrgerActStop_numb) -> GcCMS_DChrgChrgerActStop_numb/1
  3B0_1000ms/9(GcCMS_DChrgBattInsulationErr_numb) -> GcCMS_DChrgBattInsulationErr_numb/1
  3B0_1000ms/10(GcCMS_DChrgOutpCnntOvrTempErr_numb) -> GcCMS_DChrgOutpCnntOvrTempErr_numb/1
  3B0_1000ms/11(GcCMS_PcbOvrTempErr_numb) -> GcCMS_PcbOvrTempErr_numb/1
  3B0_1000ms/12(GcCMS_ChrgCnntErr_numb) -> GcCMS_ChrgCnntErr_numb/1
  3B0_1000ms/13(GcCMS_BattOvrTempErr_numb) -> GcCMS_BattOvrTempErr_numb/1
  3B0_1000ms/14(GcCMS_MainRelayErr_numb) -> GcCMS_MainRelayErr_numb/1
  3B0_1000ms/15(GcCMS_CC2ChkVoltErr_numb) -> GcCMS_CC2ChkVoltErr_numb/1
  3B0_1000ms/16(GcCMS_OtherErr_numb) -> GcCMS_OtherErr_numb/1
  3B0_1000ms/17(GcCMS_ChrgCurrAbnrm_numb) -> GcCMS_ChrgCurrAbnrm_numb/1
  3B0_1000ms/18(GcCMS_ChrgVoltAbnrm_numb) -> GcCMS_ChrgVoltAbnrm_numb/1
  3E0_20ms/1(GcCMS_CellVoltCnt_numb) -> GcCMS_CellVoltCnt_numb/1
  3E0_20ms/2(GcCMS_CellVolt1_V) -> GcCMS_CellVolt1_V/1
  3E0_20ms/3(GcCMS_CellVolt2_V) -> GcCMS_CellVolt2_V/1
  3E0_20ms/4(GcCMS_CellVolt3_V) -> GcCMS_CellVolt3_V/1
  3E0_20ms/5(GcCMS_CellVolt4_V) -> GcCMS_CellVolt4_V/1
  3E1_100ms/1(GcCMS_CellTempCnt_numb) -> GcCMS_CellTempCnt_numb/1
  3E1_100ms/2(GcCMS_CellTemp1_C) -> GcCMS_CellTemp1_C/1
  3E1_100ms/3(GcCMS_CellTemp2_C) -> GcCMS_CellTemp2_C/1
  3E1_100ms/4(GcCMS_CellTemp3_C) -> GcCMS_CellTemp3_C/1
  3E1_100ms/5(GcCMS_CellTemp4_C) -> GcCMS_CellTemp4_C/1
  3E1_100ms/6(GcCMS_CellTemp5_C) -> GcCMS_CellTemp5_C/1
  3E1_100ms/7(GcCMS_CellTemp6_C) -> GcCMS_CellTemp6_C/1
  3E1_100ms/8(GcCMS_CellTemp7_C) -> GcCMS_CellTemp7_C/1
  GeCTC_CtrCtlState_enum/1 -> Bus Creator/1  "GeCTC_CtrCtlState_enum"
  GbCTC_NegCtlState_flg/1 -> Bus Creator/2  "GbCTC_NegCtlState_flg"
  GbCTC_PosCtlState_flg/1 -> Bus Creator/3  "GbCTC_PosCtlState_flg"
  GbCTC_DCPosChrgCtlState_flg/1 -> Bus Creator/4  "GbCTC_DCPosChrgCtlState_flg"
  GbCTC_DCNegChrgCtlState_flg/1 -> Bus Creator/5  "GbCTC_DCNegChrgCtlState_flg"
  GcHDP_PackVolt_V/1 -> Bus Creator/6  "GcHDP_PackVolt_V"
  GbCTC_PreChrgCtlState_flg/1 -> Bus Creator/7  "GbCTC_PreChrgCtlState_flg"
  GcHDP_PackCrnt_A/1 -> Bus Creator/8  "GcHDP_PackCrnt_A"
  GbWSM_Kl15WkUpPrs_flg/1 -> Bus Creator/9  "GbWSM_Kl15WkUpPrs_flg"
  GcCDP_MinCellVolt_mV/1 -> Bus Creator/10  "GcCDP_MinCellVolt_mV"
  GcCDP_MaxCellVolt_mV/1 -> Bus Creator/11  "GcCDP_MaxCellVolt_mV"
  GbACC_ObcChrgCmd_flg/1 -> Bus Creator/12  "GbACC_ObcChrgCmd_flg"
  GcACC_ACChrgVoltRqst_V/1 -> Bus Creator/13  "GcACC_ACChrgVoltRqst_V"
  GcACC_ACChrgCrntRqst_A/1 -> Bus Creator/14  "GcACC_ACChrgCrntRqst_A"
  GbACC_ACChrgRqst_flg/1 -> Bus Creator/15  "GbACC_ACChrgRqst_flg"
  GeCTC_CtrCtlConnMode_enum/1 -> Bus Creator/16  "GeCTC_CtrCtlConnMode_enum"
  GbMSM_SelfCheck_flg/1 -> Bus Creator/17  "GbMSM_SelfCheck_flg"
  GcSOC_DispSOC_pct/1 -> Bus Creator/18  "GcSOC_DispSOC_pct"
  GbISP_TFHvilLFlt_flg/1 -> Bus Creator/19  "GbISP_TFHvilLFlt_flg"
  GbFTC_OpenContactor_flg/1 -> Bus Creator/20  "GbFTC_OpenContactor_flg"
  GcSOH_PackSOH_pct/1 -> Bus Creator/21  "GcSOH_PackSOH_pct"
  GcSOC_PackSOC_pct/1 -> Bus Creator/22  "GcSOC_PackSOC_pct"
  GcHDP_HallCrnt_A/1 -> Bus Creator/23  "GcHDP_HallCrnt_A"
  GbMSM_SelfChckMaxTiReach_flg/1 -> Bus Creator/24  "GbMSM_SelfChckMaxTiReach_flg"
  GaCDP_CellBalc_flg/1 -> Bus Creator/25  "GaCDP_CellBalc_flg"
  GbDCC_DCChrgRqst_flg/1 -> Bus Creator/26  "GbDCC_DCChrgRqst_flg"
  GcSOP_DischrgConstPwr_kW/1 -> Bus Creator/27  "GcSOP_DischrgConstPwr_kW"
  GcSOP_ChrgConstPwr_kW/1 -> Bus Creator/28  "GcSOP_ChrgConstPwr_kW"
  GcISO_HVIsoValue_kohm/1 -> Bus Creator/29  "GcISO_HVIsoValue_kohm"
  GeODP_ObcCcSt_enum/1 -> Bus Creator/30  "GeODP_ObcCcSt_enum"
  GbDCC_DCChrgFinish_flg/1 -> Bus Creator/31  "GbDCC_DCChrgFinish_flg"
  GbACC_ACChrgFinish_flg/1 -> Bus Creator/32  "GbACC_ACChrgFinish_flg"
  GeACC_ACChrgState_enum/1 -> Bus Creator/33  "GeACC_ACChrgState_enum"
  GeDCC_DCConnSt_enum/1 -> Bus Creator/34  "GeDCC_DCConnSt_enum"
  GeLDP_CC2St_enum/1 -> Bus Creator/35  "GeLDP_CC2St_enum"
  GcCDP_AvgCellTemp_C/1 -> Bus Creator/36  "GcCDP_AvgCellTemp_C"
  GbISO_IsoForbid_flg/1 -> Bus Creator/37  "GbISO_IsoForbid_flg"
  GcCDP_MaxCellTemp_C/1 -> Bus Creator/38  "GcCDP_MaxCellTemp_C"
  GcCDP_MinCellTemp_C/1 -> Bus Creator/39  "GcCDP_MinCellTemp_C"
  GcDCS_3072ChrgVoltReq_V/1 -> Bus Creator/40  "GcDCS_3072ChrgVoltReq_V"
  GcDCC_DCChrgCrntRqst_A/1 -> Bus Creator/41  "GcDCC_DCChrgCrntRqst_A"
  GaCDP_CellVolt_mV/1 -> Bus Creator/42  "GaCDP_CellVolt_mV"
  GaCDP_CellTemp_C/1 -> Bus Creator/43  "GaCDP_CellTemp_C"
  GcLDP_lntWtTemp_C/1 -> Bus Creator/44  "GcLDP_lntWtTemp_C"
  GcLDP_OutWtTemp_C/1 -> Bus Creator/45  "GcLDP_OutWtTemp_C"
  GcBTM_CoolPwrReq_W/1 -> Bus Creator/46  "GcBTM_CoolPwrReq_W"
  GcBTM_HeatPwrReq_W/1 -> Bus Creator/47  "GcBTM_HeatPwrReq_W"
  GeBTM_CoolReq_enum/1 -> Bus Creator/48  "GeBTM_CoolReq_enum"
  GeBTM_HeatReq_enum/1 -> Bus Creator/49  "GeBTM_HeatReq_enum"
  Bus Creator/1 -> 2CF_100msBusSelector2/1, 2CF_100msBusSelector1/1, 3B0_1000msBusSelector/1, 2CF_100msBusSelector/1, 2CE_100msBusSelector/1, 2CF_100msBusSelector3/1, 2CD_100msBusSelector/1, 2CA_100msBusSelector/1, 2C8_100msBusSelector/1, 2C0_100msBusSelector/1, 09D_10msBusSelector/1, 2C3_100msBusSelector1/1, 2C3_100msBusSelector/1, 2C7_100msBusSelector/1
  2CF_100msBusSelector1/1 -> 3E0_20ms/1(GaCDP_CellVolt_mV)  "<GaCDP_CellVolt_mV>"
  2CF_100msBusSelector2/1 -> 3E1_100ms/1(GaCDP_CellTemp_C)  "<GaCDP_CellTemp_C>"
  GbODP_V2XDischrgCmd_flg/1 -> Bus Creator/50  "GbODP_V2XDischrgCmd_flg"
  2C7_100msBusSelector/7 -> 2C7_100ms/7(GbODP_V2XDischrgCmd_flg)  "<GbODP_V2XDischrgCmd_flg>"
  GeMSM_BMUState_enum/1 -> Bus Creator/51  "GeMSM_BMUState_enum"
  2C8_100msBusSelector/8 -> 2C8_100ms/8(GeCTC_CtrCtlState_enum)  "<GeCTC_CtrCtlState_enum>"
  2C8_100msBusSelector/9 -> 2C8_100ms/9(GeMSM_BMUState_enum)  "<GeMSM_BMUState_enum>"
  2CF_100msBusSelector/5 -> 2CF_100ms/5(GcSOC_DispSOC_pct)  "<GcSOC_DispSOC_pct>"
  GcHDP_FuseVolt_V/1 -> Bus Creator/52  "GcHDP_FuseVolt_V"
  2CF_100msBusSelector/6 -> 2CF_100ms/6(GcHDP_FuseVolt_V)  "<GcHDP_FuseVolt_V>"
  2C8_100msBusSelector/10 -> 2C8_100ms/10(GeODP_ObcCcSt_enum)  "<GeODP_ObcCcSt_enum>"
  GbADP_DischgReq_flg/1 -> Bus Creator/53  "GbADP_DischgReq_flg"
  2CA_100msBusSelector/5 -> 2CA_100ms/5(GbADP_DischgReq_flg)  "<GbADP_DischgReq_flg>"
  2CA_100msBusSelector/6 -> 2CA_100ms/6(GcHDP_PackVolt_V)  "<GcHDP_PackVolt_V>"
  GcHDP_PosCtlVolt_V/1 -> Bus Creator/54  "GcHDP_PosCtlVolt_V"
  09D_10msBusSelector/9 -> 09D_10ms/9(GcHDP_PosCtlVolt_V)  "<GcHDP_PosCtlVolt_V>"
  318_500ms/5(GcCMS_MaxVoltNumb_numb) -> GcCMS_MaxVoltNumb_numb/1
  318_500ms/8(GcCMS_MinTempNumb_numb) -> GcCMS_MinTempNumb_numb/1
  318_500ms/7(GcCMS_MaxTempNumb_numb) -> GcCMS_MaxTempNumb_numb/1
  318_500ms/9(GeCMS_ChgMode_enum) -> GeCMS_ChgMode_enum/1
  318_500ms/14(GeCMS_PreThmObsvr_enum) -> GeCMS_PreThmObsvr_enum/1
  318_500ms/4(GcCMS_MinCellTempNumb_numb) -> GcCMS_MinCellTempNumb_numb/1
  318_500ms/3(GcCMS_MaxCellTempNumb_numb) -> GcCMS_MaxCellTempNumb_numb/1
  318_500ms/10(GeCMS_DChrgModeDebug_enum) -> GeCMS_DChrgModeDebug_enum/1
  318_500ms/2(GcCMS_MinCellVoltNumb_numb) -> GcCMS_MinCellVoltNumb_numb/1
  318_500ms/13(GeCMS_AChrgObsr_enum) -> GeCMS_AChrgObsr_enum/1
  318_500ms/6(GcCMS_MinVoltNumb_numb) -> GcCMS_MinVoltNumb_numb/1
  318_500ms/1(GcCMS_MaxCellVoltNumb_numb) -> GcCMS_MaxCellVoltNumb_numb/1
  318_500ms/12(GeCMS_EvccMode_enum) -> GeCMS_EvccMode_enum/1
  318_500ms/11(GbCMS_DChrgWkUp_flg) -> GbCMS_DChrgWkUp_flg/1
  GcCDP_MinCellTempNumb_numb/1 -> Bus Creator/58  "GcCDP_MinCellTempNumb_numb"
  GcCDP_MinCellVoltNumb_numb/1 -> Bus Creator/56  "GcCDP_MinCellVoltNumb_numb"
  GcCDP_MaxCellVoltNumb_numb/1 -> Bus Creator/55  "GcCDP_MaxCellVoltNumb_numb"
  GcCDP_MaxCellTempNumb_numb/1 -> Bus Creator/57  "GcCDP_MaxCellTempNumb_numb"
  GbWSM_DCWkUpPrs_flg/1 -> Bus Creator/59  "GbWSM_DCWkUpPrs_flg"
  2CF_100msBusSelector3/2 -> 318_500ms/2(GcCDP_MinCellVoltNumb_numb)  "<GcCDP_MinCellVoltNumb_numb>"
  2CF_100msBusSelector3/3 -> 318_500ms/3(GcCDP_MaxCellTempNumb_numb)  "<GcCDP_MaxCellTempNumb_numb>"
  2CF_100msBusSelector3/4 -> 318_500ms/4(GcCDP_MinCellTempNumb_numb)  "<GcCDP_MinCellTempNumb_numb>"
  2CF_100msBusSelector3/5 -> 318_500ms/5(GbWSM_DCWkUpPrs_flg)  "<GbWSM_DCWkUpPrs_flg>"
  2CF_100msBusSelector3/1 -> 318_500ms/1(GcCDP_MaxCellVoltNumb_numb)  "<GcCDP_MaxCellVoltNumb_numb>"
  GbACC_PreThmObcChrgCmd_flg/1 -> Bus Creator/60  "GbACC_PreThmObcChrgCmd_flg"
  2C7_100msBusSelector/8 -> 2C7_100ms/8(GbACC_PreThmObcChrgCmd_flg)  "<GbACC_PreThmObcChrgCmd_flg>"
  GbACC_PreHeatPrmt_flg/1 -> Bus Creator/63  "GbACC_PreHeatPrmt_flg"
  GcACC_PreThmCrntRqst_A/1 -> Bus Creator/62  "GcACC_PreThmCrntRqst_A"
  GcACC_PreThmVoltRqst_V/1 -> Bus Creator/64  "GcACC_PreThmVoltRqst_V"
  GbACC_PreThmRqst_flg/1 -> Bus Creator/61  "GbACC_PreThmRqst_flg"
  2C7_100msBusSelector/9 -> 2C7_100ms/9(GcACC_PreThmCrntRqst_A)  "<GcACC_PreThmCrntRqst_A>"
  2C7_100msBusSelector/10 -> 2C7_100ms/10(GcACC_PreThmVoltRqst_V)  "<GcACC_PreThmVoltRqst_V>"
  2C7_100msBusSelector/11 -> 2C7_100ms/11(GbACC_PreHeatPrmt_flg)  "<GbACC_PreHeatPrmt_flg>"
  2CA_100msBusSelector/7 -> 2CA_100ms/7(GbACC_PreThmRqst_flg)  "<GbACC_PreThmRqst_flg>"
  GbFTC_PowerDown_flg/1 -> Bus Creator/65  "GbFTC_PowerDown_flg"
  2CA_100msBusSelector/8 -> 2CA_100ms/8(GbFTC_PowerDown_flg)  "<GbFTC_PowerDown_flg>"
  GcBTM_CoolTempReq_C/1 -> Bus Creator/66  "GcBTM_CoolTempReq_C"
  GcBTM_HeatTempReq_C/1 -> Bus Creator/67  "GcBTM_HeatTempReq_C"
  2C3_100msBusSelector/3 -> 2C3_100ms/3(GcBTM_CoolTempReq_C)  "<GcBTM_CoolTempReq_C>"
  2C3_100msBusSelector/4 -> 2C3_100ms/4(GcBTM_HeatTempReq_C)  "<GcBTM_HeatTempReq_C>"
  2CA_100msBusSelector/9 -> 2CA_100ms/9(GbACC_PreHeatPrmt_flg)  "<GbACC_PreHeatPrmt_flg>"
  GcACC_ChrgingTiRem_min/1 -> Bus Creator/68  "GcACC_ChrgingTiRem_min"
  GcDCC_ChrgingTiRem_min/1 -> Bus Creator/69  "GcDCC_ChrgingTiRem_min"
  2CE_100msBusSelector/9 -> 2CE_100ms/9(GcACC_ChrgingTiRem_min)  "<GcACC_ChrgingTiRem_min>"
  2CE_100msBusSelector/10 -> 2CE_100ms/10(GcDCC_ChrgingTiRem_min)  "<GcDCC_ChrgingTiRem_min>"
  2CE_100msBusSelector/11 -> 2CE_100ms/11(GeCTC_CtrCtlConnMode_enum)  "<GeCTC_CtrCtlConnMode_enum>"
  GeVDP_PreThmEna_enum/1 -> Bus Creator/70  "GeVDP_PreThmEna_enum"
  2C8_100msBusSelector/11 -> 2C8_100ms/11(GeVDP_PreThmEna_enum)  "<GeVDP_PreThmEna_enum>"
  GcSOP_DischrgPwr_kW/1 -> Bus Creator/71  "GcSOP_DischrgPwr_kW"
  GcSOP_ChrgPwr_kW/1 -> Bus Creator/72  "GcSOP_ChrgPwr_kW"
  2CD_100msBusSelector/1 -> 2CD_100ms/1(GcSOP_DischrgPwr_kW)  "<GcSOP_DischrgPwr_kW>"
  2CD_100msBusSelector/2 -> 2CD_100ms/2(GcSOP_ChrgPwr_kW)  "<GcSOP_ChrgPwr_kW>"
  2CE_100msBusSelector/12 -> 2CE_100ms/12(GbACC_PreHeatPrmt_flg)  "<GbACC_PreHeatPrmt_flg>"
  2CE_100msBusSelector/13 -> 2CE_100ms/13(GeVDP_PreThmEna_enum)  "<GeVDP_PreThmEna_enum>"
  2CA_100msBusSelector/10 -> 2CA_100ms/10(GeVDP_PreThmEna_enum)  "<GeVDP_PreThmEna_enum>"
  GbFTC_DischrgPwrLimitLevel3_flg/1 -> Bus Creator/73  "GbFTC_DischrgPwrLimitLevel3_flg"
  GbFTC_RegenPwrLimitLevel1_flg/1 -> Bus Creator/80  "GbFTC_RegenPwrLimitLevel1_flg"
  GbFTC_DischrgPwrLimitLevel1_flg/1 -> Bus Creator/79  "GbFTC_DischrgPwrLimitLevel1_flg"
  GbFTC_ACChrgCurrLimitLevel2_flg/1 -> Bus Creator/78  "GbFTC_ACChrgCurrLimitLevel2_flg"
  GbFTC_DCChrgCurrLimitLevel2_flg/1 -> Bus Creator/77  "GbFTC_DCChrgCurrLimitLevel2_flg"
  GbFTC_RegenPwrLimitLevel2_flg/1 -> Bus Creator/76  "GbFTC_RegenPwrLimitLevel2_flg"
  GbFTC_DischrgPwrLimitLevel2_flg/1 -> Bus Creator/75  "GbFTC_DischrgPwrLimitLevel2_flg"
  GbFTC_RegenPwrLimitLevel3_flg/1 -> Bus Creator/74  "GbFTC_RegenPwrLimitLevel3_flg"
  2C8_100msBusSelector/12 -> 2C8_100ms/12(GbFTC_OpenContactor_flg)  "<GbFTC_OpenContactor_flg>"
  2C8_100msBusSelector/13 -> 2C8_100ms/13(GbFTC_PowerDown_flg)  "<GbFTC_PowerDown_flg>"
  2C8_100msBusSelector/14 -> 2C8_100ms/14(GbFTC_DischrgPwrLimitLevel3_flg)  "<GbFTC_DischrgPwrLimitLevel3_flg>"
  2C8_100msBusSelector/15 -> 2C8_100ms/15(GbFTC_RegenPwrLimitLevel3_flg)  "<GbFTC_RegenPwrLimitLevel3_flg>"
  2C8_100msBusSelector/16 -> 2C8_100ms/16(GbFTC_DischrgPwrLimitLevel2_flg)  "<GbFTC_DischrgPwrLimitLevel2_flg>"
  2C8_100msBusSelector/17 -> 2C8_100ms/17(GbFTC_RegenPwrLimitLevel2_flg)  "<GbFTC_RegenPwrLimitLevel2_flg>"
  2C8_100msBusSelector/18 -> 2C8_100ms/18(GbFTC_DCChrgCurrLimitLevel2_flg)  "<GbFTC_DCChrgCurrLimitLevel2_flg>"
  2C8_100msBusSelector/19 -> 2C8_100ms/19(GbFTC_ACChrgCurrLimitLevel2_flg)  "<GbFTC_ACChrgCurrLimitLevel2_flg>"
  2C8_100msBusSelector/20 -> 2C8_100ms/20(GbFTC_DischrgPwrLimitLevel1_flg)  "<GbFTC_DischrgPwrLimitLevel1_flg>"
  2C8_100msBusSelector/21 -> 2C8_100ms/21(GbFTC_RegenPwrLimitLevel1_flg)  "<GbFTC_RegenPwrLimitLevel1_flg>"
  09D_10ms/12(GeCMS_Thm_propagat_enum) -> GeCMS_Thm_propagat_enum/1
  GcCDP_MaxBusbarTemp_C/1 -> Bus Creator/81  "GcCDP_MaxBusbarTemp_C"
  GcCDP_MinBusbarTemp_C/1 -> Bus Creator/82  "GcCDP_MinBusbarTemp_C"
  2C3_100msBusSelector/5 -> 2C3_100ms/5(GcCDP_MaxBusbarTemp_C)  "<GcCDP_MaxBusbarTemp_C>"
  2C3_100msBusSelector/6 -> 2C3_100ms/6(GcCDP_MinBusbarTemp_C)  "<GcCDP_MinBusbarTemp_C>"
  2C3_100msBusSelector1/1 -> 2C2_100ms/1(GcSOP_DischrgPwr_kW)  "<GcSOP_DischrgPwr_kW>"
  2C3_100msBusSelector1/2 -> 2C2_100ms/2(GcSOP_ChrgPwr_kW)  "<GcSOP_ChrgPwr_kW>"
  2C3_100msBusSelector1/3 -> 2C2_100ms/3(GcHDP_PackVolt_V)  "<GcHDP_PackVolt_V>"
  2CA_100msBusSelector/11 -> 2CA_100ms/11(GcSOP_DischrgConstPwr_kW)  "<GcSOP_DischrgConstPwr_kW>"
  2CA_100msBusSelector/12 -> 2CA_100ms/12(GcSOP_ChrgConstPwr_kW)  "<GcSOP_ChrgConstPwr_kW>"
  GeDCC_DCChrgState_enum/1 -> Bus Creator/83  "GeDCC_DCChrgState_enum"
  2CE_100msBusSelector/14 -> 2CE_100ms/14(GeDCC_DCChrgState_enum)  "<GeDCC_DCChrgState_enum>"
  GeLDP_ChrgGunConnSt_enum/1 -> Bus Creator/84  "GeLDP_ChrgGunConnSt_enum"
  2CE_100msBusSelector/15 -> 2CE_100ms/15(GeLDP_ChrgGunConnSt_enum)  "<GeLDP_ChrgGunConnSt_enum>"
  GbISP_TFThmRnwyfDet_flg/1 -> Bus Creator/85  "GbISP_TFThmRnwyfDet_flg"
  09D_10msBusSelector/10 -> 09D_10ms/10(GbISP_TFThmRnwyfDet_flg)  "<GbISP_TFThmRnwyfDet_flg>"
  09D_10ms/13(GbCMS_StartCanSend_flg) -> GbCMS_StartCanSend_flg/1
  GcUDS_CellTempNumb_numb/1 -> Bus Creator/87  "GcUDS_CellTempNumb_numb"
  GcUDS_BusbarTempNumb_numb/1 -> Bus Creator/88  "GcUDS_BusbarTempNumb_numb"
  GaCDP_BusbarTemp_C/1 -> Bus Creator/86  "GaCDP_BusbarTemp_C"
  2CF_100msBusSelector2/2 -> 3E1_100ms/2(GaCDP_BusbarTemp_C)  "<GaCDP_BusbarTemp_C>"
  2CF_100msBusSelector2/3 -> 3E1_100ms/3(GcUDS_CellTempNumb_numb)  "<GcUDS_CellTempNumb_numb>"
  2CF_100msBusSelector2/4 -> 3E1_100ms/4(GcUDS_BusbarTempNumb_numb)  "<GcUDS_BusbarTempNumb_numb>"
  GcUDS_CellVoltNum_numb/1 -> Bus Creator/89  "GcUDS_CellVoltNum_numb"
  2CF_100msBusSelector1/2 -> 3E0_20ms/2(GcUDS_CellVoltNum_numb)  "<GcUDS_CellVoltNum_numb>"
  GcUDS_BatEnergy_kWh/1 -> Bus Creator/90  "GcUDS_BatEnergy_kWh"
  2CF_100msBusSelector/7 -> 2CF_100ms/7(GcUDS_BatEnergy_kWh)  "<GcUDS_BatEnergy_kWh>"
  GbACC_HoldTempPrmt_flg/1 -> Bus Creator/91  "GbACC_HoldTempPrmt_flg"
  GbACC_HoldTempObcChrgCmd_flg/1 -> Bus Creator/92  "GbACC_HoldTempObcChrgCmd_flg"
  GcACC_HoldTempVoltRqst_V/1 -> Bus Creator/93  "GcACC_HoldTempVoltRqst_V"
  GcACC_HoldTempCrntRqst_A/1 -> Bus Creator/94  "GcACC_HoldTempCrntRqst_A"
  GbACC_HoldTempRqst_flg/1 -> Bus Creator/95  "GbACC_HoldTempRqst_flg"
  2C7_100msBusSelector/12 -> 2C7_100ms/12(GbACC_HoldTempObcChrgCmd_flg)  "<GbACC_HoldTempObcChrgCmd_flg>"
  2C7_100msBusSelector/13 -> 2C7_100ms/13(GbACC_HoldTempPrmt_flg)  "<GbACC_HoldTempPrmt_flg>"
  2C7_100msBusSelector/14 -> 2C7_100ms/14(GcACC_HoldTempVoltRqst_V)  "<GcACC_HoldTempVoltRqst_V>"
  2C7_100msBusSelector/15 -> 2C7_100ms/15(GcACC_HoldTempCrntRqst_A)  "<GcACC_HoldTempCrntRqst_A>"
  2CA_100msBusSelector/13 -> 2CA_100ms/13(GbACC_HoldTempPrmt_flg)  "<GbACC_HoldTempPrmt_flg>"
  2CA_100msBusSelector/14 -> 2CA_100ms/14(GbACC_HoldTempRqst_flg)  "<GbACC_HoldTempRqst_flg>"
  2C8_100ms/13(GeCMS_AppChgMode_enum) -> GeCMS_AppChgMode_enum/1
  GbISP_TFIsoResFltLevel2_flg/1 -> Bus Creator/96  "GbISP_TFIsoResFltLevel2_flg"
  GbISP_TFIsoDCResFltLevel2_flg/1 -> Bus Creator/97  "GbISP_TFIsoDCResFltLevel2_flg"
  GbISP_TFIsoHVoffResFltLevel2_flg/1 -> Bus Creator/98  "GbISP_TFIsoHVoffResFltLevel2_flg"
  GbISP_TFIsoResFltLevel1_flg/1 -> Bus Creator/99  "GbISP_TFIsoResFltLevel1_flg"
  GbISP_TFIsoDCResFltLevel1_flg/1 -> Bus Creator/100  "GbISP_TFIsoDCResFltLevel1_flg"
  GbISP_TFIsoHVoffResFltLevel1_flg/1 -> Bus Creator/101  "GbISP_TFIsoHVoffResFltLevel1_flg"
  2C8_100msBusSelector/22 -> 2C8_100ms/22(GbISP_TFIsoResFltLevel2_flg)  "<GbISP_TFIsoResFltLevel2_flg>"
  2C8_100msBusSelector/23 -> 2C8_100ms/23(GbISP_TFIsoDCResFltLevel2_flg)  "<GbISP_TFIsoDCResFltLevel2_flg>"
  2C8_100msBusSelector/24 -> 2C8_100ms/24(GbISP_TFIsoHVoffResFltLevel2_flg)  "<GbISP_TFIsoHVoffResFltLevel2_flg>"
  2C8_100msBusSelector/25 -> 2C8_100ms/25(GbISP_TFIsoResFltLevel1_flg)  "<GbISP_TFIsoResFltLevel1_flg>"
  2C8_100msBusSelector/26 -> 2C8_100ms/26(GbISP_TFIsoDCResFltLevel1_flg)  "<GbISP_TFIsoDCResFltLevel1_flg>"
  2C8_100msBusSelector/27 -> 2C8_100ms/27(GbISP_TFIsoHVoffResFltLevel1_flg)  "<GbISP_TFIsoHVoffResFltLevel1_flg>"
  GbFTC_Level1FltReaction_flg/1 -> Bus Creator/102  "GbFTC_Level1FltReaction_flg"
  2C8_100msBusSelector/28 -> 2C8_100ms/28(GbFTC_Level1FltReaction_flg)  "<GbFTC_Level1FltReaction_flg>"
  2C3_100msBusSelector/7 -> 2C3_100ms/7(GcUDS_BusbarTempNumb_numb)  "<GcUDS_BusbarTempNumb_numb>"
  2C3_100msBusSelector/8 -> 2C3_100ms/8(GcCDP_MaxCellTemp_C)  "<GcCDP_MaxCellTemp_C>"
  2C3_100msBusSelector/9 -> 2C3_100ms/9(GcCDP_MinCellTemp_C)  "<GcCDP_MinCellTemp_C>"
  2CF_100msBusSelector/8 -> 2CF_100ms/8(GcUDS_CellTempNumb_numb)  "<GcUDS_CellTempNumb_numb>"
  2CF_100msBusSelector/9 -> 2CF_100ms/9(GcCDP_MaxBusbarTemp_C)  "<GcCDP_MaxBusbarTemp_C>"
  2CF_100msBusSelector/10 -> 2CF_100ms/10(GcCDP_MinBusbarTemp_C)  "<GcCDP_MinBusbarTemp_C>"

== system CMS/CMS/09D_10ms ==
  GeCTC_CtrCtlState_enum : Inport
  GbCTC_NegCtlState_flg : Inport  Port=2
  GbCTC_PosCtlState_flg : Inport  Port=3
  GbCTC_DCPosChrgCtlState_flg : Inport  Port=4
  GbCTC_DCNegChrgCtlState_flg : Inport  Port=5
  GbCTC_PreChrgCtlState_flg : Inport  Port=6
  GcHDP_PackCrnt_A : Inport  Port=7
  GbWSM_Kl15WkUpPrs_flg : Inport  Port=8
  GcHDP_PosCtlVolt_V : Inport  Port=9
  GbISP_TFThmRnwyfDet_flg : Inport  Port=10
  CMS_09D_10ms : TriggerPort  TriggerType=function-call  VariantControl=(inherit)
  09D_10ms_sys : Subsystem
  GeCMS_HVConnSt_enum : Outport
  GbCMS_NegCtlSt_flg : Outport  Port=2
  GbCMS_PosCtlSt_flg : Outport  Port=3
  GbCMS_ChrgPosCtlSt_flg : Outport  Port=4
  GbCMS_ChrgNegCtlSt_flg : Outport  Port=5
  GeCMS_RelStuckClosed_enum : Outport  Port=6
  GcCMS_PackVolt_V : Outport  Port=7
  GbCMS_PreChrgCtlSt_flg : Outport  Port=8
  GcCMS_BattCurr_A : Outport  Port=9
  GbCMS_Kl15WkUp_flg : Outport  Port=10
  GbCMS_ThmRunAway_flg : Outport  Port=11
  GeCMS_Thm_propagat_enum : Outport  Port=12
  GbCMS_StartCanSend_flg : Outport  Port=13
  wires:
  GeCTC_CtrCtlState_enum/1 -> 09D_10ms_sys/1(GeCTC_CtrCtlState_enum)
  GbCTC_NegCtlState_flg/1 -> 09D_10ms_sys/2(GbCTC_NegCtlState_flg)
  GbCTC_PosCtlState_flg/1 -> 09D_10ms_sys/3(GbCTC_PosCtlState_flg)
  GbCTC_DCPosChrgCtlState_flg/1 -> 09D_10ms_sys/4(GbCTC_DCPosChrgCtlState_flg)
  GbCTC_DCNegChrgCtlState_flg/1 -> 09D_10ms_sys/5(GbCTC_DCNegChrgCtlState_flg)
  GcHDP_PosCtlVolt_V/1 -> 09D_10ms_sys/9(GcHDP_PosCtlVolt_V)
  GbCTC_PreChrgCtlState_flg/1 -> 09D_10ms_sys/6(GbCTC_PreChrgCtlState_flg)
  GcHDP_PackCrnt_A/1 -> 09D_10ms_sys/7(GcHDP_PackCrnt_A)
  GbWSM_Kl15WkUpPrs_flg/1 -> 09D_10ms_sys/8(GbWSM_Kl15WkUpPrs_flg)
  09D_10ms_sys/1(GeCMS_HVConnSt_enum) -> GeCMS_HVConnSt_enum/1
  09D_10ms_sys/2(GbCMS_NegCtlSt_flg) -> GbCMS_NegCtlSt_flg/1
  09D_10ms_sys/3(GbCMS_PosCtlSt_flg) -> GbCMS_PosCtlSt_flg/1
  09D_10ms_sys/4(GbCMS_ChrgPosCtlSt_flg) -> GbCMS_ChrgPosCtlSt_flg/1
  09D_10ms_sys/5(GbCMS_ChrgNegCtlSt_flg) -> GbCMS_ChrgNegCtlSt_flg/1
  09D_10ms_sys/6(GeCMS_RelStuckClosed_enum) -> GeCMS_RelStuckClosed_enum/1
  09D_10ms_sys/7(GcCMS_PackVolt_V) -> GcCMS_PackVolt_V/1
  09D_10ms_sys/8(GbCMS_PreChrgCtlSt_flg) -> GbCMS_PreChrgCtlSt_flg/1
  09D_10ms_sys/9(GcCMS_BattCurr_A) -> GcCMS_BattCurr_A/1
  09D_10ms_sys/10(GbCMS_Kl15WkUp_flg) -> GbCMS_Kl15WkUp_flg/1
  09D_10ms_sys/11(GbCMS_ThmRunAway_flg) -> GbCMS_ThmRunAway_flg/1
  09D_10ms_sys/12(GeCMS_Thm_propagat_enum) -> GeCMS_Thm_propagat_enum/1
  GbISP_TFThmRnwyfDet_flg/1 -> 09D_10ms_sys/10(GbISP_TFThmRnwyfDet_flg)
  09D_10ms_sys/13(GbCMS_StartCanSend_flg) -> GbCMS_StartCanSend_flg/1

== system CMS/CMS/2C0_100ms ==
  GcLDP_lntWtTemp_C : Inport
  GcLDP_OutWtTemp_C : Inport  Port=2
  GcBTM_CoolPwrReq_W : Inport  Port=3
  GcBTM_HeatPwrReq_W : Inport  Port=4
  GeBTM_CoolReq_enum : Inport  Port=5
  GeBTM_HeatReq_enum : Inport  Port=6
  CMS_2C0_100ms : TriggerPort  TriggerType=function-call  VariantControl=(inherit)
  2C0_100ms_sys : Subsystem
  GcCMS_CoolTempIn_C : Outport
  GcCMS_CoolTempOut_C : Outport  Port=2
  GcCMS_CoolPwrReq_W : Outport  Port=3
  GcCMS_HeatPwrReq_W : Outport  Port=4
  GeCMS_CoolReq_enum : Outport  Port=5
  GeCMS_HeatReq_enum : Outport  Port=6
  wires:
  GcLDP_lntWtTemp_C/1 -> 2C0_100ms_sys/1(GcLDP_lntWtTemp_C)
  GcLDP_OutWtTemp_C/1 -> 2C0_100ms_sys/2(GcLDP_OutWtTemp_C)
  GcBTM_CoolPwrReq_W/1 -> 2C0_100ms_sys/3(GcBTM_CoolPwrReq_W)
  GcBTM_HeatPwrReq_W/1 -> 2C0_100ms_sys/4(GcBTM_HeatPwrReq_W)
  GeBTM_CoolReq_enum/1 -> 2C0_100ms_sys/5(GeBTM_CoolReq_enum)
  GeBTM_HeatReq_enum/1 -> 2C0_100ms_sys/6(GeBTM_HeatReq_enum)
  2C0_100ms_sys/1(GcCMS_CoolTempIn_C) -> GcCMS_CoolTempIn_C/1
  2C0_100ms_sys/2(GcCMS_CoolTempOut_C) -> GcCMS_CoolTempOut_C/1
  2C0_100ms_sys/3(GcCMS_CoolPwrReq_W) -> GcCMS_CoolPwrReq_W/1
  2C0_100ms_sys/4(GcCMS_HeatPwrReq_W) -> GcCMS_HeatPwrReq_W/1
  2C0_100ms_sys/5(GeCMS_CoolReq_enum) -> GeCMS_CoolReq_enum/1
  2C0_100ms_sys/6(GeCMS_HeatReq_enum) -> GeCMS_HeatReq_enum/1

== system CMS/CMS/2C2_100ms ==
  GcSOP_DischrgPwr_kW : Inport
  GcSOP_ChrgPwr_kW : Inport  Port=2
  GcHDP_PackVolt_V : Inport  Port=3
  CMS_2C2_100ms : TriggerPort  TriggerType=function-call  VariantControl=(inherit)
  2C2_100ms_sys : Subsystem
  GcCMS_PeakCurrDisCh_A : Outport
  GcCMS_PeakCurrCh_A : Outport  Port=2
  GcCMS_PeakVoltDisCh_V : Outport  Port=3
  GcCMS_PeakVoltCh_V : Outport  Port=4
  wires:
  2C2_100ms_sys/1(GcCMS_PeakCurrDisCh_A) -> GcCMS_PeakCurrDisCh_A/1
  2C2_100ms_sys/2(GcCMS_PeakCurrCh_A) -> GcCMS_PeakCurrCh_A/1
  2C2_100ms_sys/3(GcCMS_PeakVoltDisCh_V) -> GcCMS_PeakVoltDisCh_V/1
  2C2_100ms_sys/4(GcCMS_PeakVoltCh_V) -> GcCMS_PeakVoltCh_V/1
  GcSOP_DischrgPwr_kW/1 -> 2C2_100ms_sys/1(GcSOP_DischrgPwr_kW)
  GcSOP_ChrgPwr_kW/1 -> 2C2_100ms_sys/2(GcSOP_ChrgPwr_kW)
  GcHDP_PackVolt_V/1 -> 2C2_100ms_sys/3(GcHDP_PackVolt_V)
